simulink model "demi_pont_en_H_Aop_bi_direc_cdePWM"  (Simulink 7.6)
settings: Solver=ode15s  StartTime=0.0  StopTime=0.3  RelTol=1e-3
InitFcn:
  | clc
  | delete *.mat
StopFcn:
  | close all, clc
  | load demi_pont_en_H_bi_direct.mat
  | subplot 211
  | plotyy(x(1,:),x(4,:),x(1,:),x(3,:))
  | xlabel('temps')
  | title('Position et vitesse angulaires - Moteur CC, 1/2 Pont en H bidirectionnel - Cde PWM')
  | grid
  | %axis([0 N -0.2 1.2])
  | subplot 212
  | plot(x(1,:),x(2,:))
  | delete *.mat
libraries: fl_lib x25, nesl_utility x18, elec_lib x15

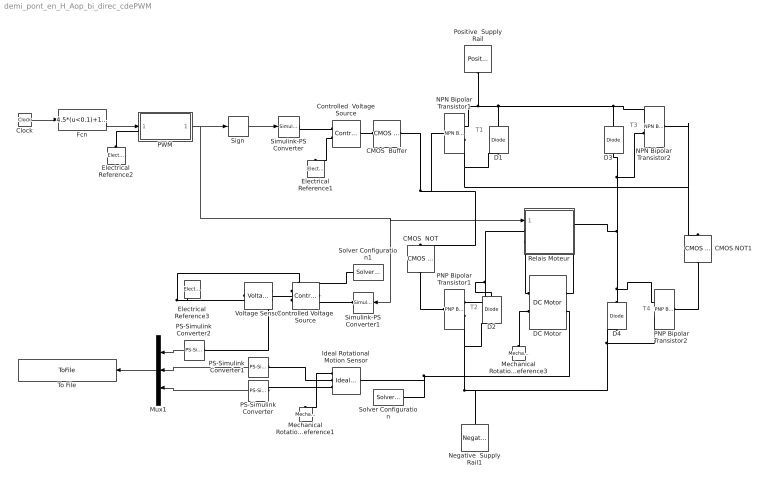
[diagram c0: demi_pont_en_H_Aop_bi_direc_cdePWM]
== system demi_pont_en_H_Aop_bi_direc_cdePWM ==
  note: T1
  note: T4
  note: T3
  note: T2
  CMOS  Buffer : elec_lib/Integrated Circuits/Logic/CMOS Buffer  DialogController=NetworkEngine.DynNeDlgSource  SystemSampleTime=-1  V_IL=2 V  V_IH=3 V  C_IN=5 pF  output_type=1  V_OL=0 V  V_OH=5 V  V_CC=5 V  V_meas=5 V  R_OUT=25 Ohm  R_OH=[ 25 250 ] Ohm  I_OH=63 mA  R_OL=[ 30 800 ] Ohm  I_OL=-45 mA  Delay=25 ns  Ron=5 Ohm  Vf=0.6 V  output_state=1  LocalVarLogging=[]
  CMOS  NOT : elec_lib/Integrated Circuits/Logic/CMOS NOT  DialogController=NetworkEngine.DynNeDlgSource  SystemSampleTime=-1  V_IL=2 V  V_IH=3 V  C_IN=5 pF  output_type=1  V_OL=0 V  V_OH=5 V  V_CC=5 V  V_meas=5 V  R_OUT=25 Ohm  R_OH=[ 25 250 ] Ohm  I_OH=63 mA  R_OL=[ 30 800 ] Ohm  I_OL=-45 mA  Delay=25 ns  Ron=5 Ohm  Vf=0.6 V  output_state=1  LocalVarLogging=[]
  CMOS NOT1 : elec_lib/Integrated Circuits/Logic/CMOS NOT  DialogController=NetworkEngine.DynNeDlgSource  SystemSampleTime=-1  V_IL=2 V  V_IH=3 V  C_IN=5 pF  output_type=1  V_OL=0 V  V_OH=5 V  V_CC=5 V  V_meas=5 V  R_OUT=25 Ohm  R_OH=[ 25 250 ] Ohm  I_OH=63 mA  R_OL=[ 30 800 ] Ohm  I_OL=-45 mA  Delay=25 ns  Ron=5 Ohm  Vf=0.6 V  output_state=1  LocalVarLogging=[]
  Clock : Clock
  Controlled  Voltage Source : fl_lib/Electrical/Electrical Sources/Controlled Voltage Source  DialogController=NetworkEngine.DynNeDlgSource  SystemSampleTime=-1  i_Log=off  v_Log=off  LocalVarNames=|i|v  LocalVarDescs=|i|v  LocalVarLogging=[0 0]
  Controlled Voltage Source : fl_lib/Electrical/Electrical Sources/Controlled Voltage Source  DialogController=NetworkEngine.DynNeDlgSource  SystemSampleTime=-1  i_Log=off  v_Log=off  LocalVarNames=|i|v  LocalVarDescs=|i|v  LocalVarLogging=[0 0]
  D{1..4} (4 alike) : elec_lib/Semiconductor Devices/Diode  DialogController=NetworkEngine.DynNeDlgSource  SystemSampleTime=-1  ModelType=1  Vf=0.6 V  Ron=0.3 Ohm  Goff=1e-8 S  Rz=0.3 Ohm  Vz=50 V  C_PWL=5 pF  prmExp=1  I12=[ 0.07 1.5 ] A  V12=[ 0.7 0.8 ] V  I1=0.07 A  V1=0.7 V  RS=0.01 Ohm  IS=1e-14 A  Tmeas=25 C  ec=1  BV=Inf V  C_param=1  CJ0=5 pF  VJ=1 V  Mgrad=0.5  Vvec=[ 0.1 10 100 ] V  Cvec=[ 3.5 1 0.4 ] pF  FC=0.5  LocalVarLogging=[]
  DC Motor : elec_lib/Actuators & Drivers/Rotational Actuators/DC Motor  DialogController=NetworkEngine.DynNeDlgSource  SystemSampleTime=-1  parameterization=1  Ra=3.9 Ohm  La=1.2e-5 H  emf_or_torque=1  Kv=7.2e-5 V/rpm  Ki=6.876e-4 N*m/A  T_stall=2.4e-4 N*m  w_max=1.91e+4 rpm  w_rated=1.5e+4 rpm  P_rated=0.08 W  V_rated=1.5 V  J=0.01 g*cm^2  lam=1e-8 N*m/(rad/s)  speed0=0.5 rpm  current_Log=off  voltage_Log=off  power_Log=off  i2r_Log=off  torque_Log=off  speed_Log=off  LocalVarNames=|current|voltage|power|i2r|torque|speed  LocalVarDescs=|Current (A)|Voltage (V)|Power (W)|Electrical losses (W)|Torque (Nm)|Angular speed (rad/s)  LocalVarLogging=[0 0 0 0 0 0]
  Electrical Reference1 : fl_lib/Electrical/Electrical Elements/Electrical Reference  DialogController=NetworkEngine.DynNeDlgSource  SystemSampleTime=-1  i_Log=off  LocalVarNames=|i  LocalVarDescs=|i  LocalVarLogging=[]
  Electrical Reference2 : fl_lib/Electrical/Electrical Elements/Electrical Reference  DialogController=NetworkEngine.DynNeDlgSource  SystemSampleTime=-1  i_Log=off  LocalVarNames=|i  LocalVarDescs=|i  LocalVarLogging=[]
  Electrical Reference3 : fl_lib/Electrical/Electrical Elements/Electrical Reference  DialogController=NetworkEngine.DynNeDlgSource  SystemSampleTime=-1  i_Log=off  LocalVarNames=|i  LocalVarDescs=|i  LocalVarLogging=[]
  Fcn : Fcn  Expr=4.5*(u<0.1)+1.5*((u>0.1)&&(u<0.2))+2.5*(u>0.2)
  Ideal Rotational Motion Sensor : fl_lib/Mechanical/Mechanical Sensors/Ideal Rotational Motion Sensor  DialogController=NetworkEngine.DynNeDlgSource  SystemSampleTime=-1  offset=0 rad  w_Log=off  t_Log=off  phi_Log=off  LocalVarNames=|w|t|phi  LocalVarDescs=|w|t|phi  LocalVarLogging=[0 0 0]
  Mechanical Rotational Reference1 : fl_lib/Mechanical/Rotational Elements/Mechanical Rotational Reference  DialogController=NetworkEngine.DynNeDlgSource  SystemSampleTime=-1  t_Log=off  LocalVarNames=|t  LocalVarDescs=|t  LocalVarLogging=0
  Mechanical Rotational Reference3 : fl_lib/Mechanical/Rotational Elements/Mechanical Rotational Reference  DialogController=NetworkEngine.DynNeDlgSource  SystemSampleTime=-1  t_Log=off  LocalVarNames=|t  LocalVarDescs=|t  LocalVarLogging=0
  Mux1 : Mux  Inputs=3
  NPN Bipolar Transistor1 : elec_lib/Semiconductor Devices/NPN Bipolar Transistor  DialogController=NetworkEngine.DynNeDlgSource  SystemSampleTime=-1  parameterization=1  BF=100  IS=1e-14 A  VAF=200 V  hfe=100  hoe=5e-5 1/Ohm  Ic_h=1 mA  V1=0.55 V  I1=0.5 mA  BR=1  Tmeas=25 C  RC=0.01 Ohm  RE=1e-4 Ohm  RB=1 Ohm  C_BC=5 pF  C_BE=5 pF  TF=0 us  TR=0 us  LocalVarLogging=[]
  NPN Bipolar Transistor2 : elec_lib/Semiconductor Devices/NPN Bipolar Transistor  DialogController=NetworkEngine.DynNeDlgSource  SystemSampleTime=-1  parameterization=1  BF=100  IS=1e-14 A  VAF=200 V  hfe=100  hoe=5e-5 1/Ohm  Ic_h=1 mA  V1=0.55 V  I1=0.5 mA  BR=1  Tmeas=25 C  RC=0.01 Ohm  RE=1e-4 Ohm  RB=1 Ohm  C_BC=5 pF  C_BE=5 pF  TF=0 us  TR=0 us  LocalVarLogging=[]
  Negative  Supply Rail1 : elec_lib/Sources/Negative Supply Rail  DialogController=NetworkEngine.DynNeDlgSource  SystemSampleTime=-1  v0=-24 V  current_Log=off  voltage_Log=off  power_Log=off  LocalVarNames=|current|voltage|power  LocalVarDescs=|Current (A)|Voltage (V)|Power (W)  LocalVarLogging=[0 0 0]
  PNP Bipolar Transistor1 : elec_lib/Semiconductor Devices/PNP Bipolar Transistor  DialogController=NetworkEngine.DynNeDlgSource  SystemSampleTime=-1  parameterization=1  BF=100  IS=1e-14 A  VAF=200 V  hfe=100  hoe=5e-5 1/Ohm  Ic_h=1 mA  V1=0.55 V  I1=0.5 mA  BR=1  Tmeas=25 C  RC=0.01 Ohm  RE=1e-4 Ohm  RB=1 Ohm  C_BC=5 pF  C_BE=5 pF  TF=0 us  TR=0 us  LocalVarLogging=[]
  PNP Bipolar Transistor2 : elec_lib/Semiconductor Devices/PNP Bipolar Transistor  DialogController=NetworkEngine.DynNeDlgSource  SystemSampleTime=-1  parameterization=1  BF=100  IS=1e-14 A  VAF=200 V  hfe=100  hoe=5e-5 1/Ohm  Ic_h=1 mA  V1=0.55 V  I1=0.5 mA  BR=1  Tmeas=25 C  RC=0.01 Ohm  RE=1e-4 Ohm  RB=1 Ohm  C_BC=5 pF  C_BE=5 pF  TF=0 us  TR=0 us  LocalVarLogging=[]
  PS-Simulink Converter : nesl_utility/PS-Simulink Converter  DialogController=NetworkEngine.DynNeUtilDlgSource  SystemSampleTime=-1  PhysicalDomain=network_engine_domain  LeftPortType=input  RightPortType=output  SubClassName=ps_output  Unit=1  AffineConversion=off
  PS-Simulink Converter1 : nesl_utility/PS-Simulink Converter  DialogController=NetworkEngine.DynNeUtilDlgSource  SystemSampleTime=-1  PhysicalDomain=network_engine_domain  LeftPortType=input  RightPortType=output  SubClassName=ps_output  Unit=1  AffineConversion=off
  PS-Simulink Converter2 : nesl_utility/PS-Simulink Converter  DialogController=NetworkEngine.DynNeUtilDlgSource  SystemSampleTime=-1  PhysicalDomain=network_engine_domain  LeftPortType=input  RightPortType=output  SubClassName=ps_output  Unit=1  AffineConversion=off
  PWM : Subsystem
  Positive  Supply Rail : elec_lib/Sources/Positive Supply Rail  DialogController=NetworkEngine.DynNeDlgSource  SystemSampleTime=-1  v0=24 V  current_Log=off  voltage_Log=off  power_Log=off  LocalVarNames=|current|voltage|power  LocalVarDescs=|Current (A)|Voltage (V)|Power (W)  LocalVarLogging=[0 0 0]
  Relais Moteur : Subsystem
  Sign : Signum
  Simulink-PS Converter : nesl_utility/Simulink-PS Converter  DialogController=NetworkEngine.DynNeUtilDlgSource  SystemSampleTime=-1  PhysicalDomain=network_engine_domain  LeftPortType=input  RightPortType=output  SubClassName=ps_input  Unit=1  AffineConversion=off  InputFilterTimeConstant=.001  UdotUserProvided=0
  Simulink-PS Converter1 : nesl_utility/Simulink-PS Converter  DialogController=NetworkEngine.DynNeUtilDlgSource  SystemSampleTime=-1  PhysicalDomain=network_engine_domain  LeftPortType=input  RightPortType=output  SubClassName=ps_input  Unit=1  AffineConversion=off  InputFilterTimeConstant=.001  UdotUserProvided=0
  Solver Configuration : nesl_utility/Solver Configuration  DialogController=NetworkEngine.DynNeUtilDlgSource  SystemSampleTime=-1  PhysicalDomain=network_engine_domain  LeftPortType=input  RightPortType=generic  SubClassName=solver  Accelerate=off  Profile=off  ResidualTolerance=1e-9  MaxNonlinIter=3  MaxModeIter=2  DoFixedCost=off  UseLocalSampling=off  DoDC=off  LinearAlgebra=Sparse  LocalSolverSampleTime=.001  LocalSolverChoice=NE_BACKWARD_EULER_ADVANCER  UseLocalSolver=off
  Solver Configuration1 : nesl_utility/Solver Configuration  DialogController=NetworkEngine.DynNeUtilDlgSource  SystemSampleTime=-1  PhysicalDomain=network_engine_domain  LeftPortType=input  RightPortType=generic  SubClassName=solver  Accelerate=off  Profile=off  ResidualTolerance=1e-9  MaxNonlinIter=3  MaxModeIter=2  DoFixedCost=off  UseLocalSampling=off  DoDC=off  LinearAlgebra=Sparse  LocalSolverSampleTime=.001  LocalSolverChoice=NE_BACKWARD_EULER_ADVANCER  UseLocalSolver=off
  To File : ToFile  Filename=demi_pont_en_H_bi_direct  MatrixName=x
  Voltage Sensor : fl_lib/Electrical/Electrical Sensors/Voltage Sensor  DialogController=NetworkEngine.DynNeDlgSource  SystemSampleTime=-1  i1_Log=off  v1_Log=off  LocalVarNames=|i1|v1  LocalVarDescs=|i1|v1  LocalVarLogging=[0 0]
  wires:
  Mux1/1 -> To File/1
  PWM/1(PWM) -> Sign/1, Relais Moteur/1(cde_sens), Simulink-PS Converter1/1
  Sign/1 -> Simulink-PS Converter/1
  PS-Simulink Converter/1 -> Mux1/3
  PS-Simulink Converter1/1 -> Mux1/2
  PS-Simulink Converter2/1 -> Mux1/1
  Fcn/1 -> PWM/1(+ref)
  Clock/1 -> Fcn/1
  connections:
  D3/RConn1 -- NPN Bipolar Transistor2/RConn1 -- Positive  Supply Rail/RConn1 -- NPN Bipolar Transistor1/RConn1 -- D1/RConn1
  CMOS  Buffer/LConn1 -- Controlled  Voltage Source/LConn1
  Simulink-PS Converter/RConn1 -- Controlled  Voltage Source/RConn1
  Relais Moteur/LConn1 -- PNP Bipolar Transistor1/RConn1 -- D2/RConn1
  Controlled  Voltage Source/RConn2 -- Electrical Reference1/LConn1
  D4/RConn1 -- PNP Bipolar Transistor2/RConn1 -- Relais Moteur/RConn1 -- D3/LConn1 -- NPN Bipolar Transistor2/RConn2
  Relais Moteur/LConn2 -- DC Motor/RConn1
  Relais Moteur/RConn2 -- DC Motor/LConn1
  Mechanical Rotational Reference3/LConn1 -- DC Motor/RConn2
  PNP Bipolar Transistor1/RConn2 -- Negative  Supply Rail1/LConn1 -- D4/LConn1 -- PNP Bipolar Transistor2/RConn2 -- D2/LConn1
  PS-Simulink Converter/LConn1 -- Ideal Rotational Motion Sensor/RConn3
  Ideal Rotational Motion Sensor/RConn1 -- Mechanical Rotational Reference1/LConn1
  DC Motor/LConn2 -- Ideal Rotational Motion Sensor/LConn1 -- Solver Configuration/RConn1
  NPN Bipolar Transistor1/RConn2 -- NPN Bipolar Transistor1/LConn1 -- CMOS  Buffer/RConn1 -- CMOS  NOT/LConn1 -- CMOS NOT1/LConn1 -- NPN Bipolar Transistor2/LConn1 -- D1/LConn1
  CMOS  NOT/RConn1 -- PNP Bipolar Transistor1/LConn1
  CMOS NOT1/RConn1 -- PNP Bipolar Transistor2/LConn1
  Electrical Reference2/LConn1 -- PWM/LConn1
  Ideal Rotational Motion Sensor/RConn2 -- PS-Simulink Converter1/LConn1
  Controlled Voltage Source/RConn1 -- Simulink-PS Converter1/RConn1
  Voltage Sensor/RConn1 -- PS-Simulink Converter2/LConn1
  Voltage Sensor/LConn1 -- Controlled Voltage Source/LConn1
  Controlled Voltage Source/RConn2 -- Electrical Reference3/LConn1 -- Voltage Sensor/RConn2 -- Solver Configuration1/RConn1

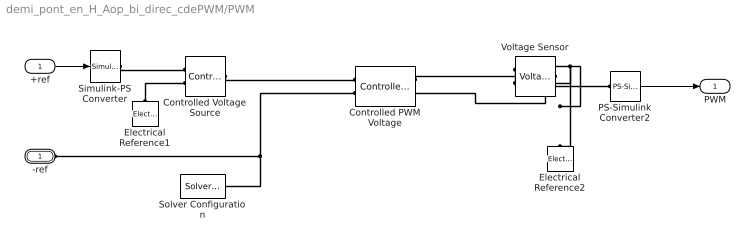
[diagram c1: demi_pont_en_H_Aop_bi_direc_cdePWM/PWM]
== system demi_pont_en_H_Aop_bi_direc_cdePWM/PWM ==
  +ref : Inport
  Controlled PWM Voltage : elec_lib/Actuators & Drivers/Drivers/Controlled PWM Voltage  DialogController=NetworkEngine.DynNeDlgSource  SystemSampleTime=-1  F=10000 Hz  Vmin=0 V  Vmax=5 V  Vm=5 V  pwm_or_av=1  current_Log=off  voltage_Log=off  power_Log=off  LocalVarNames=|current|voltage|power  LocalVarDescs=|Load current (A)|Load voltage (V)|Load power (W)  LocalVarLogging=[0 0 0]
  Controlled Voltage Source : fl_lib/Electrical/Electrical Sources/Controlled Voltage Source  DialogController=NetworkEngine.DynNeDlgSource  SystemSampleTime=-1  i_Log=off  v_Log=off  LocalVarNames=|i|v  LocalVarDescs=|i|v  LocalVarLogging=[0 0]
  Electrical Reference1 : fl_lib/Electrical/Electrical Elements/Electrical Reference  DialogController=NetworkEngine.DynNeDlgSource  SystemSampleTime=-1  i_Log=off  LocalVarNames=|i  LocalVarDescs=|i  LocalVarLogging=[]
  Electrical Reference2 : fl_lib/Electrical/Electrical Elements/Electrical Reference  DialogController=NetworkEngine.DynNeDlgSource  SystemSampleTime=-1  i_Log=off  LocalVarNames=|i  LocalVarDescs=|i  LocalVarLogging=[]
  PS-Simulink Converter2 : nesl_utility/PS-Simulink Converter  DialogController=NetworkEngine.DynNeUtilDlgSource  SystemSampleTime=-1  PhysicalDomain=network_engine_domain  LeftPortType=input  RightPortType=output  SubClassName=ps_output  Unit=1  AffineConversion=off
  Simulink-PS Converter : nesl_utility/Simulink-PS Converter  DialogController=NetworkEngine.DynNeUtilDlgSource  SystemSampleTime=-1  PhysicalDomain=network_engine_domain  LeftPortType=input  RightPortType=output  SubClassName=ps_input  Unit=1  AffineConversion=off  InputFilterTimeConstant=.001  UdotUserProvided=0
  Solver Configuration : nesl_utility/Solver Configuration  DialogController=NetworkEngine.DynNeUtilDlgSource  SystemSampleTime=-1  PhysicalDomain=network_engine_domain  LeftPortType=input  RightPortType=generic  SubClassName=solver  Accelerate=off  Profile=off  ResidualTolerance=1e-9  MaxNonlinIter=3  MaxModeIter=2  DoFixedCost=off  UseLocalSampling=off  DoDC=off  LinearAlgebra=Sparse  LocalSolverSampleTime=.001  LocalSolverChoice=NE_BACKWARD_EULER_ADVANCER  UseLocalSolver=off
  Voltage Sensor : fl_lib/Electrical/Electrical Sensors/Voltage Sensor  DialogController=NetworkEngine.DynNeDlgSource  SystemSampleTime=-1  i1_Log=off  v1_Log=off  LocalVarNames=|i1|v1  LocalVarDescs=|i1|v1  LocalVarLogging=[0 0]
  -ref : PMIOPort  Port=1  Side=Left
  PWM : Outport
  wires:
  PS-Simulink Converter2/1 -> PWM/1
  +ref/1 -> Simulink-PS Converter/1
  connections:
  -ref/RConn1 -- Controlled PWM Voltage/LConn2 -- Solver Configuration/RConn1
  Controlled PWM Voltage/RConn1 -- Voltage Sensor/LConn1
  Voltage Sensor/RConn2 -- Controlled PWM Voltage/RConn2 -- Electrical Reference2/LConn1
  Voltage Sensor/RConn1 -- PS-Simulink Converter2/LConn1
  Controlled Voltage Source/LConn1 -- Controlled PWM Voltage/LConn1
  Electrical Reference1/LConn1 -- Controlled Voltage Source/RConn2
  Simulink-PS Converter/RConn1 -- Controlled Voltage Source/RConn1

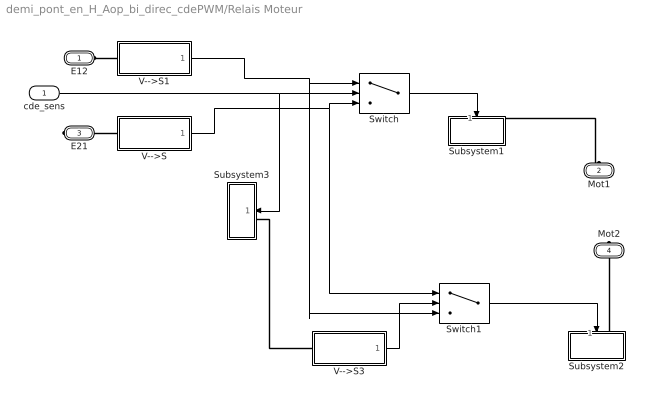
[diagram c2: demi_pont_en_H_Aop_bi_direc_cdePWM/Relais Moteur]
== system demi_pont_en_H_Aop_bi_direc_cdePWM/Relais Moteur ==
  cde_sens : Inport
  Subsystem1 : Subsystem
  Subsystem2 : Subsystem
  Subsystem3 : Subsystem
  Switch : Switch  Threshold=0.5
  Switch1 : Switch  Threshold=0.5
  V-->S : Subsystem
  V-->S1 : Subsystem
  V-->S3 : Subsystem
  E12 : PMIOPort  Port=1  Side=Left
  Mot1 : PMIOPort  Port=2  Side=Left
  E21 : PMIOPort  Port=3  Side=Right
  Mot2 : PMIOPort  Port=4  Side=Right
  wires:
  V-->S/1(S) -> Switch/3, Switch1/1
  V-->S1/1(S) -> Switch/1, Switch1/3
  V-->S3/1(S) -> Switch1/2
  Switch/1 -> Subsystem1/1(S)
  cde_sens/1 -> Switch/2, Subsystem3/1(S)
  Switch1/1 -> Subsystem2/1(S)
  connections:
  Subsystem1/LConn1 -- Mot1/RConn1
  Subsystem3/LConn1 -- V-->S3/LConn1
  E12/RConn1 -- V-->S1/LConn1
  E21/RConn1 -- V-->S/LConn1
  Mot2/RConn1 -- Subsystem2/LConn1

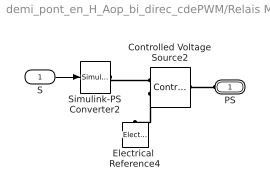
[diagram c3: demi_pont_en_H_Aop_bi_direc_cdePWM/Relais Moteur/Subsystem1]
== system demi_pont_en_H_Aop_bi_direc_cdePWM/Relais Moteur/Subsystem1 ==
  S : Inport
  Controlled Voltage Source2 : fl_lib/Electrical/Electrical Sources/Controlled Voltage Source  DialogController=NetworkEngine.DynNeDlgSource  SystemSampleTime=-1  i_Log=off  v_Log=off  LocalVarNames=|i|v  LocalVarDescs=|i|v  LocalVarLogging=[0 0]
  Electrical  Reference4 : fl_lib/Electrical/Electrical Elements/Electrical Reference  DialogController=NetworkEngine.DynNeDlgSource  SystemSampleTime=-1  i_Log=off  LocalVarNames=|i  LocalVarDescs=|i  LocalVarLogging=0
  Simulink-PS Converter2 : nesl_utility/Simulink-PS Converter  DialogController=NetworkEngine.DynNeUtilDlgSource  SystemSampleTime=-1  PhysicalDomain=network_engine_domain  LeftPortType=input  RightPortType=output  SubClassName=ps_input  Unit=1  AffineConversion=off  InputFilterTimeConstant=.001  UdotUserProvided=0
  PS : PMIOPort  Port=1  Side=Left
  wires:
  S/1 -> Simulink-PS Converter2/1
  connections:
  PS/RConn1 -- Controlled Voltage Source2/LConn1
  Controlled Voltage Source2/RConn2 -- Electrical  Reference4/LConn1
  Simulink-PS Converter2/RConn1 -- Controlled Voltage Source2/RConn1

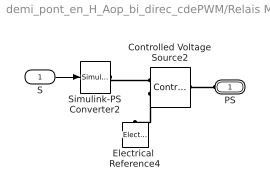
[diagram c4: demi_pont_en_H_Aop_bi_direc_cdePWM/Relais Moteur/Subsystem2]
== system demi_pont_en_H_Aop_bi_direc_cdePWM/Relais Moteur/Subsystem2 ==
  S : Inport
  Controlled Voltage Source2 : fl_lib/Electrical/Electrical Sources/Controlled Voltage Source  DialogController=NetworkEngine.DynNeDlgSource  SystemSampleTime=-1  i_Log=off  v_Log=off  LocalVarNames=|i|v  LocalVarDescs=|i|v  LocalVarLogging=[0 0]
  Electrical  Reference4 : fl_lib/Electrical/Electrical Elements/Electrical Reference  DialogController=NetworkEngine.DynNeDlgSource  SystemSampleTime=-1  i_Log=off  LocalVarNames=|i  LocalVarDescs=|i  LocalVarLogging=0
  Simulink-PS Converter2 : nesl_utility/Simulink-PS Converter  DialogController=NetworkEngine.DynNeUtilDlgSource  SystemSampleTime=-1  PhysicalDomain=network_engine_domain  LeftPortType=input  RightPortType=output  SubClassName=ps_input  Unit=1  AffineConversion=off  InputFilterTimeConstant=.001  UdotUserProvided=0
  PS : PMIOPort  Port=1  Side=Left
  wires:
  S/1 -> Simulink-PS Converter2/1
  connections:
  Simulink-PS Converter2/RConn1 -- Controlled Voltage Source2/RConn1
  Controlled Voltage Source2/RConn2 -- Electrical  Reference4/LConn1
  PS/RConn1 -- Controlled Voltage Source2/LConn1

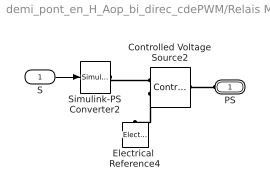
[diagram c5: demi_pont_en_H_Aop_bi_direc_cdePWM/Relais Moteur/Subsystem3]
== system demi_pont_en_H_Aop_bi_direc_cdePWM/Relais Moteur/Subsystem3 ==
  S : Inport
  Controlled Voltage Source2 : fl_lib/Electrical/Electrical Sources/Controlled Voltage Source  DialogController=NetworkEngine.DynNeDlgSource  SystemSampleTime=-1  i_Log=off  v_Log=off  LocalVarNames=|i|v  LocalVarDescs=|i|v  LocalVarLogging=[0 0]
  Electrical  Reference4 : fl_lib/Electrical/Electrical Elements/Electrical Reference  DialogController=NetworkEngine.DynNeDlgSource  SystemSampleTime=-1  i_Log=off  LocalVarNames=|i  LocalVarDescs=|i  LocalVarLogging=0
  Simulink-PS Converter2 : nesl_utility/Simulink-PS Converter  DialogController=NetworkEngine.DynNeUtilDlgSource  SystemSampleTime=-1  PhysicalDomain=network_engine_domain  LeftPortType=input  RightPortType=output  SubClassName=ps_input  Unit=1  AffineConversion=off  InputFilterTimeConstant=.001  UdotUserProvided=0
  PS : PMIOPort  Port=1  Side=Left
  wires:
  S/1 -> Simulink-PS Converter2/1
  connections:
  PS/RConn1 -- Controlled Voltage Source2/LConn1
  Controlled Voltage Source2/RConn2 -- Electrical  Reference4/LConn1
  Simulink-PS Converter2/RConn1 -- Controlled Voltage Source2/RConn1

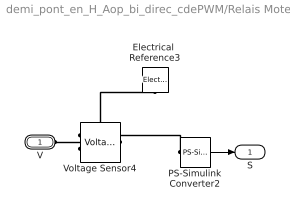
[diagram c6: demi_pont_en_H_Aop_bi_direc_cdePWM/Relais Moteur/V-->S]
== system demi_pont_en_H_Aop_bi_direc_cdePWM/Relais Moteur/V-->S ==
  Electrical  Reference3 : fl_lib/Electrical/Electrical Elements/Electrical Reference  DialogController=NetworkEngine.DynNeDlgSource  SystemSampleTime=-1  i_Log=off  LocalVarNames=|i  LocalVarDescs=|i  LocalVarLogging=0
  PS-Simulink Converter2 : nesl_utility/PS-Simulink Converter  DialogController=NetworkEngine.DynNeUtilDlgSource  SystemSampleTime=-1  PhysicalDomain=network_engine_domain  LeftPortType=input  RightPortType=output  SubClassName=ps_output  Unit=1  AffineConversion=off
  Voltage Sensor4 : fl_lib/Electrical/Electrical Sensors/Voltage Sensor  DialogController=NetworkEngine.DynNeDlgSource  SystemSampleTime=-1  i1_Log=off  v1_Log=off  LocalVarNames=|i1|v1  LocalVarDescs=|i1|v1  LocalVarLogging=[0 0]
  V : PMIOPort  Port=1  Side=Left
  S : Outport
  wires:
  PS-Simulink Converter2/1 -> S/1
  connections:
  Voltage Sensor4/RConn2 -- Electrical  Reference3/LConn1
  PS-Simulink Converter2/LConn1 -- Voltage Sensor4/RConn1
  V/RConn1 -- Voltage Sensor4/LConn1

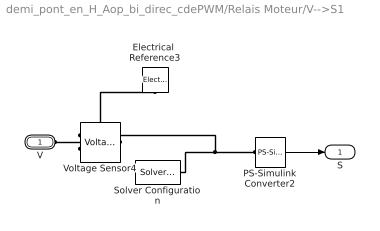
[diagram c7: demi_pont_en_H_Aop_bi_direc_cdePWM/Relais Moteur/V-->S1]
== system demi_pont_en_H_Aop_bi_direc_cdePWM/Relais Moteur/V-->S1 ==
  Electrical  Reference3 : fl_lib/Electrical/Electrical Elements/Electrical Reference  DialogController=NetworkEngine.DynNeDlgSource  SystemSampleTime=-1  i_Log=off  LocalVarNames=|i  LocalVarDescs=|i  LocalVarLogging=0
  PS-Simulink Converter2 : nesl_utility/PS-Simulink Converter  DialogController=NetworkEngine.DynNeUtilDlgSource  SystemSampleTime=-1  PhysicalDomain=network_engine_domain  LeftPortType=input  RightPortType=output  SubClassName=ps_output  Unit=1  AffineConversion=off
  Solver Configuration : nesl_utility/Solver Configuration  DialogController=NetworkEngine.DynNeUtilDlgSource  SystemSampleTime=-1  PhysicalDomain=network_engine_domain  LeftPortType=input  RightPortType=generic  SubClassName=solver  Accelerate=off  Profile=off  ResidualTolerance=1e-9  MaxNonlinIter=3  MaxModeIter=2  DoFixedCost=off  UseLocalSampling=off  DoDC=off  LinearAlgebra=Sparse  LocalSolverSampleTime=.001  LocalSolverChoice=NE_BACKWARD_EULER_ADVANCER  UseLocalSolver=off
  Voltage Sensor4 : fl_lib/Electrical/Electrical Sensors/Voltage Sensor  DialogController=NetworkEngine.DynNeDlgSource  SystemSampleTime=-1  i1_Log=off  v1_Log=off  LocalVarNames=|i1|v1  LocalVarDescs=|i1|v1  LocalVarLogging=[0 0]
  V : PMIOPort  Port=1  Side=Left
  S : Outport
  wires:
  PS-Simulink Converter2/1 -> S/1
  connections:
  V/RConn1 -- Voltage Sensor4/LConn1
  PS-Simulink Converter2/LConn1 -- Voltage Sensor4/RConn1 -- Solver Configuration/RConn1
  Voltage Sensor4/RConn2 -- Electrical  Reference3/LConn1

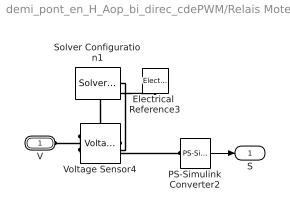
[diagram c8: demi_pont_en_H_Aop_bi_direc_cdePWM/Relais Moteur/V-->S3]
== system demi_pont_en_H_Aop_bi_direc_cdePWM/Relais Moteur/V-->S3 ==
  Electrical  Reference3 : fl_lib/Electrical/Electrical Elements/Electrical Reference  DialogController=NetworkEngine.DynNeDlgSource  SystemSampleTime=-1  i_Log=off  LocalVarNames=|i  LocalVarDescs=|i  LocalVarLogging=0
  PS-Simulink Converter2 : nesl_utility/PS-Simulink Converter  DialogController=NetworkEngine.DynNeUtilDlgSource  SystemSampleTime=-1  PhysicalDomain=network_engine_domain  LeftPortType=input  RightPortType=output  SubClassName=ps_output  Unit=1  AffineConversion=off
  Solver Configuration1 : nesl_utility/Solver Configuration  DialogController=NetworkEngine.DynNeUtilDlgSource  SystemSampleTime=-1  PhysicalDomain=network_engine_domain  LeftPortType=input  RightPortType=generic  SubClassName=solver  Accelerate=off  Profile=off  ResidualTolerance=1e-9  MaxNonlinIter=3  MaxModeIter=2  DoFixedCost=off  UseLocalSampling=off  DoDC=off  LinearAlgebra=Sparse  LocalSolverSampleTime=.001  LocalSolverChoice=NE_BACKWARD_EULER_ADVANCER  UseLocalSolver=off
  Voltage Sensor4 : fl_lib/Electrical/Electrical Sensors/Voltage Sensor  DialogController=NetworkEngine.DynNeDlgSource  SystemSampleTime=-1  i1_Log=off  v1_Log=off  LocalVarNames=|i1|v1  LocalVarDescs=|i1|v1  LocalVarLogging=[0 0]
  V : PMIOPort  Port=1  Side=Left
  S : Outport
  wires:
  PS-Simulink Converter2/1 -> S/1
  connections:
  Voltage Sensor4/RConn2 -- Electrical  Reference3/LConn1 -- Solver Configuration1/RConn1
  Voltage Sensor4/RConn1 -- PS-Simulink Converter2/LConn1
  V/RConn1 -- Voltage Sensor4/LConn1
